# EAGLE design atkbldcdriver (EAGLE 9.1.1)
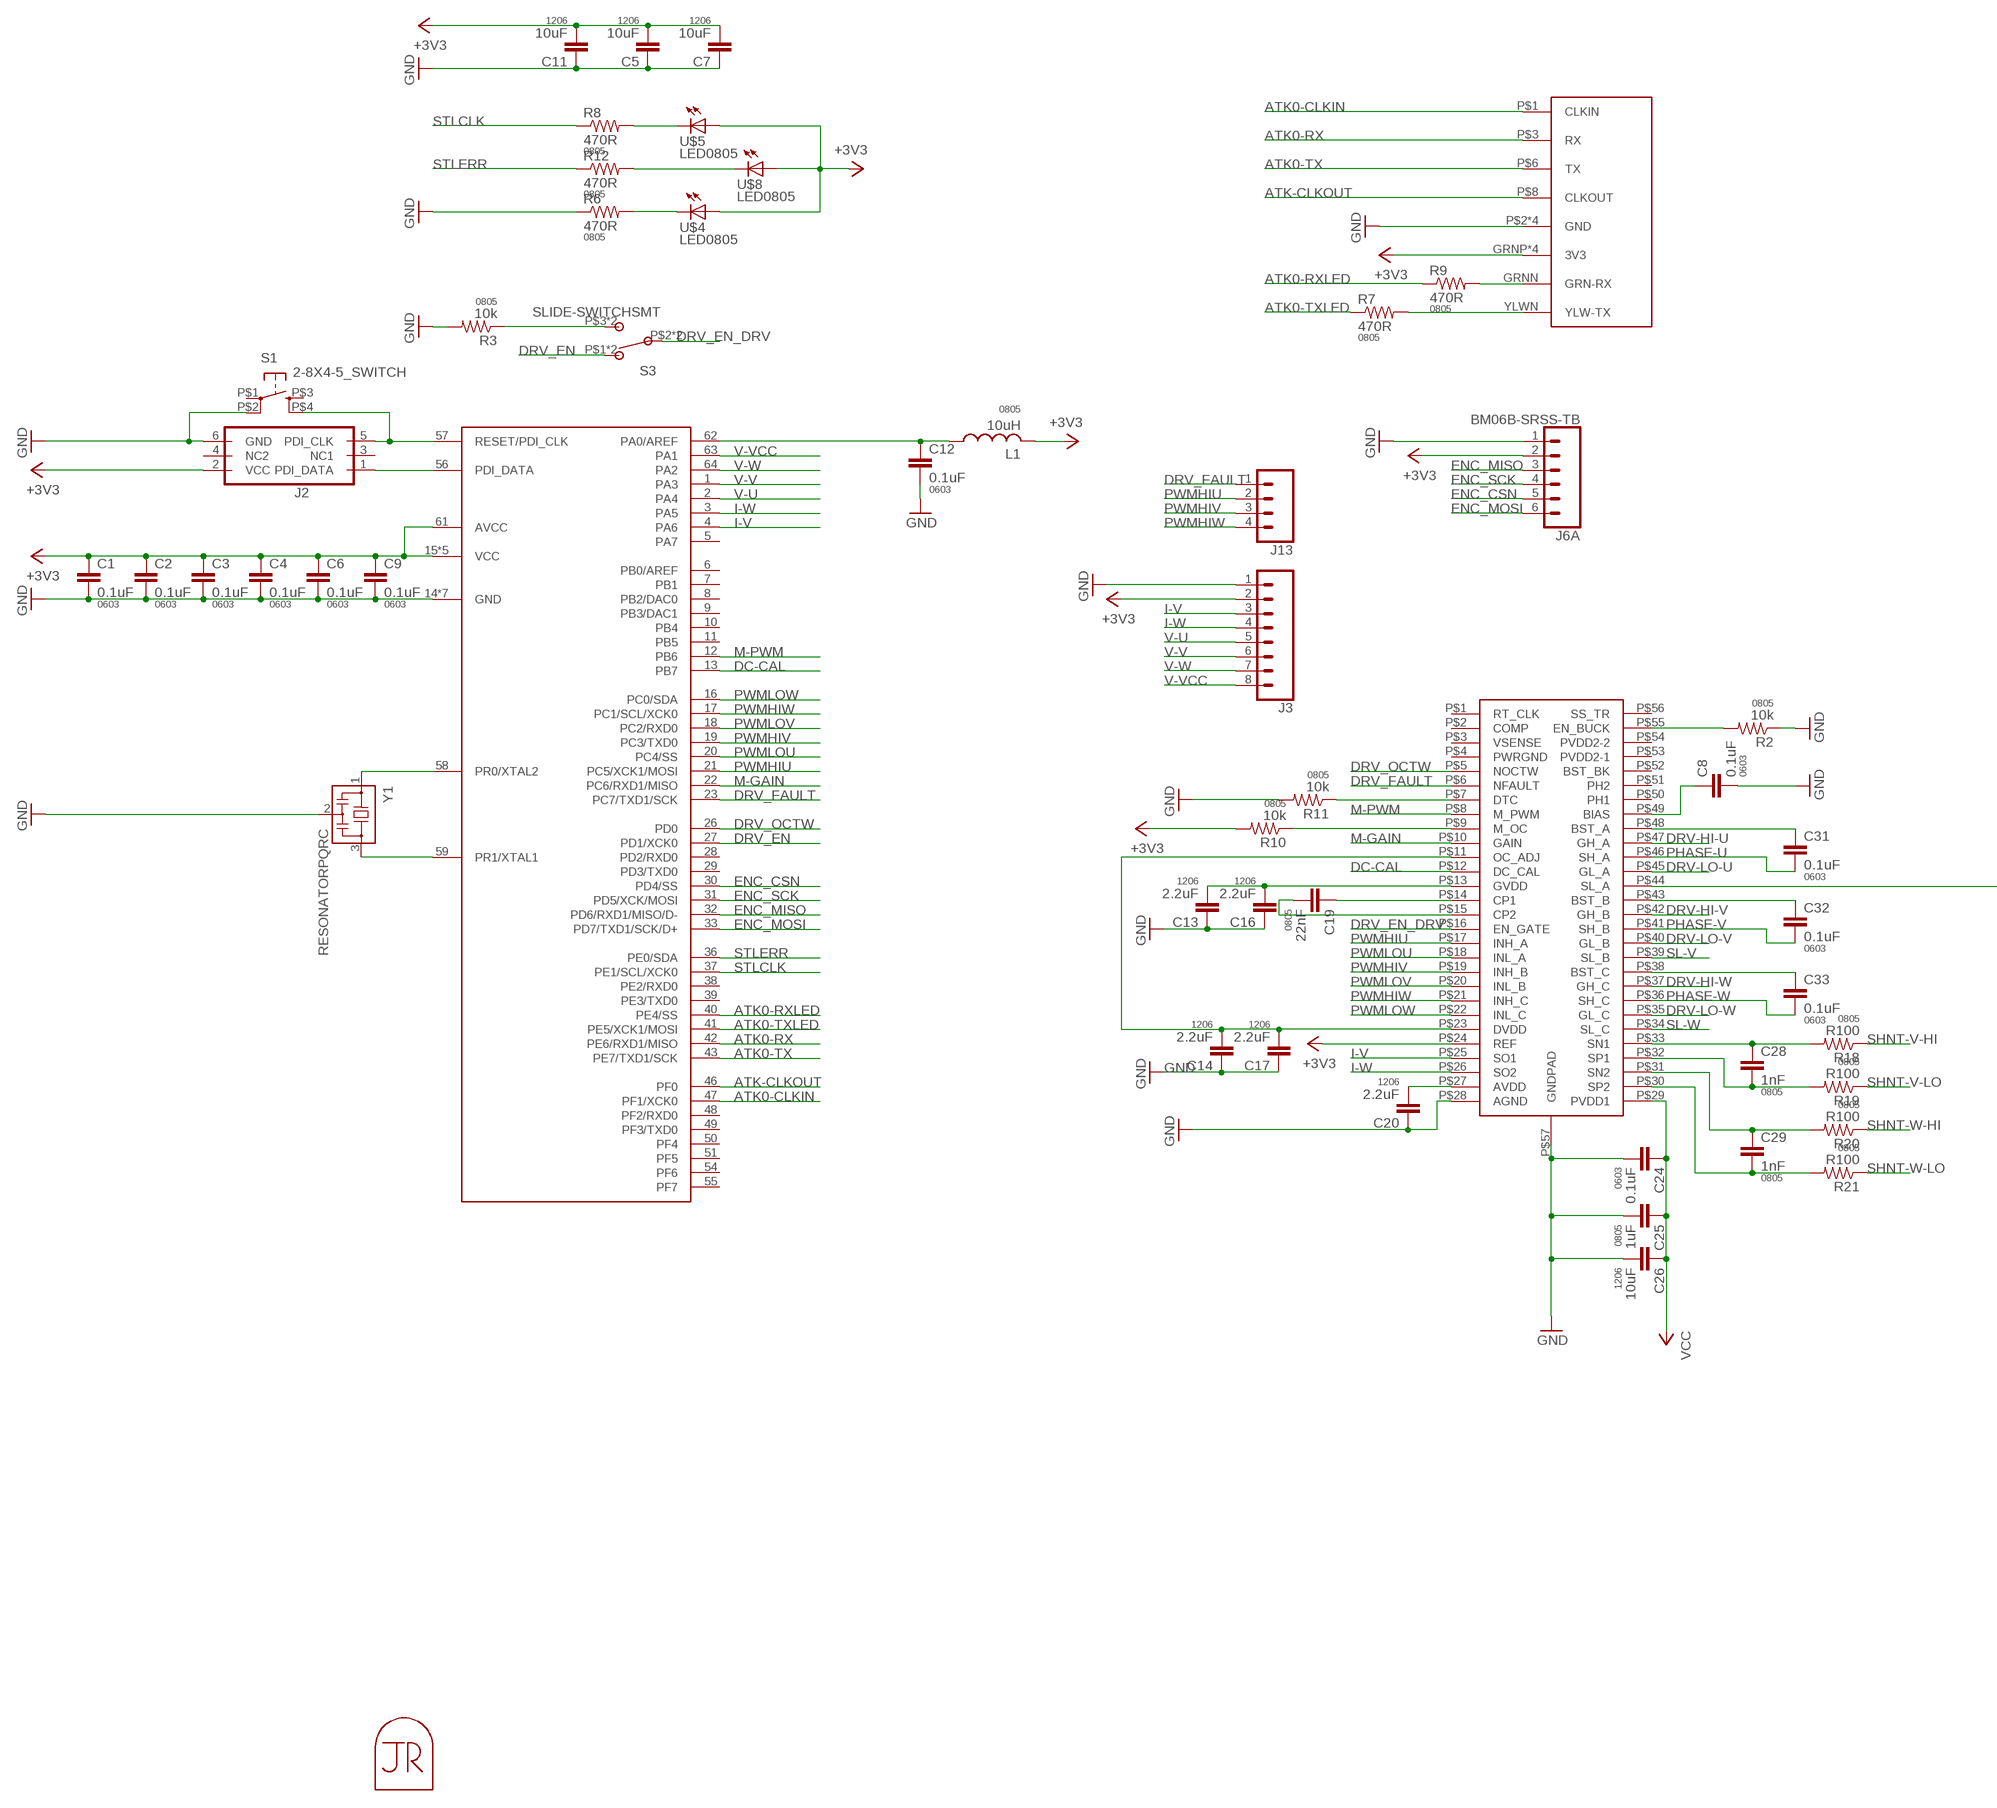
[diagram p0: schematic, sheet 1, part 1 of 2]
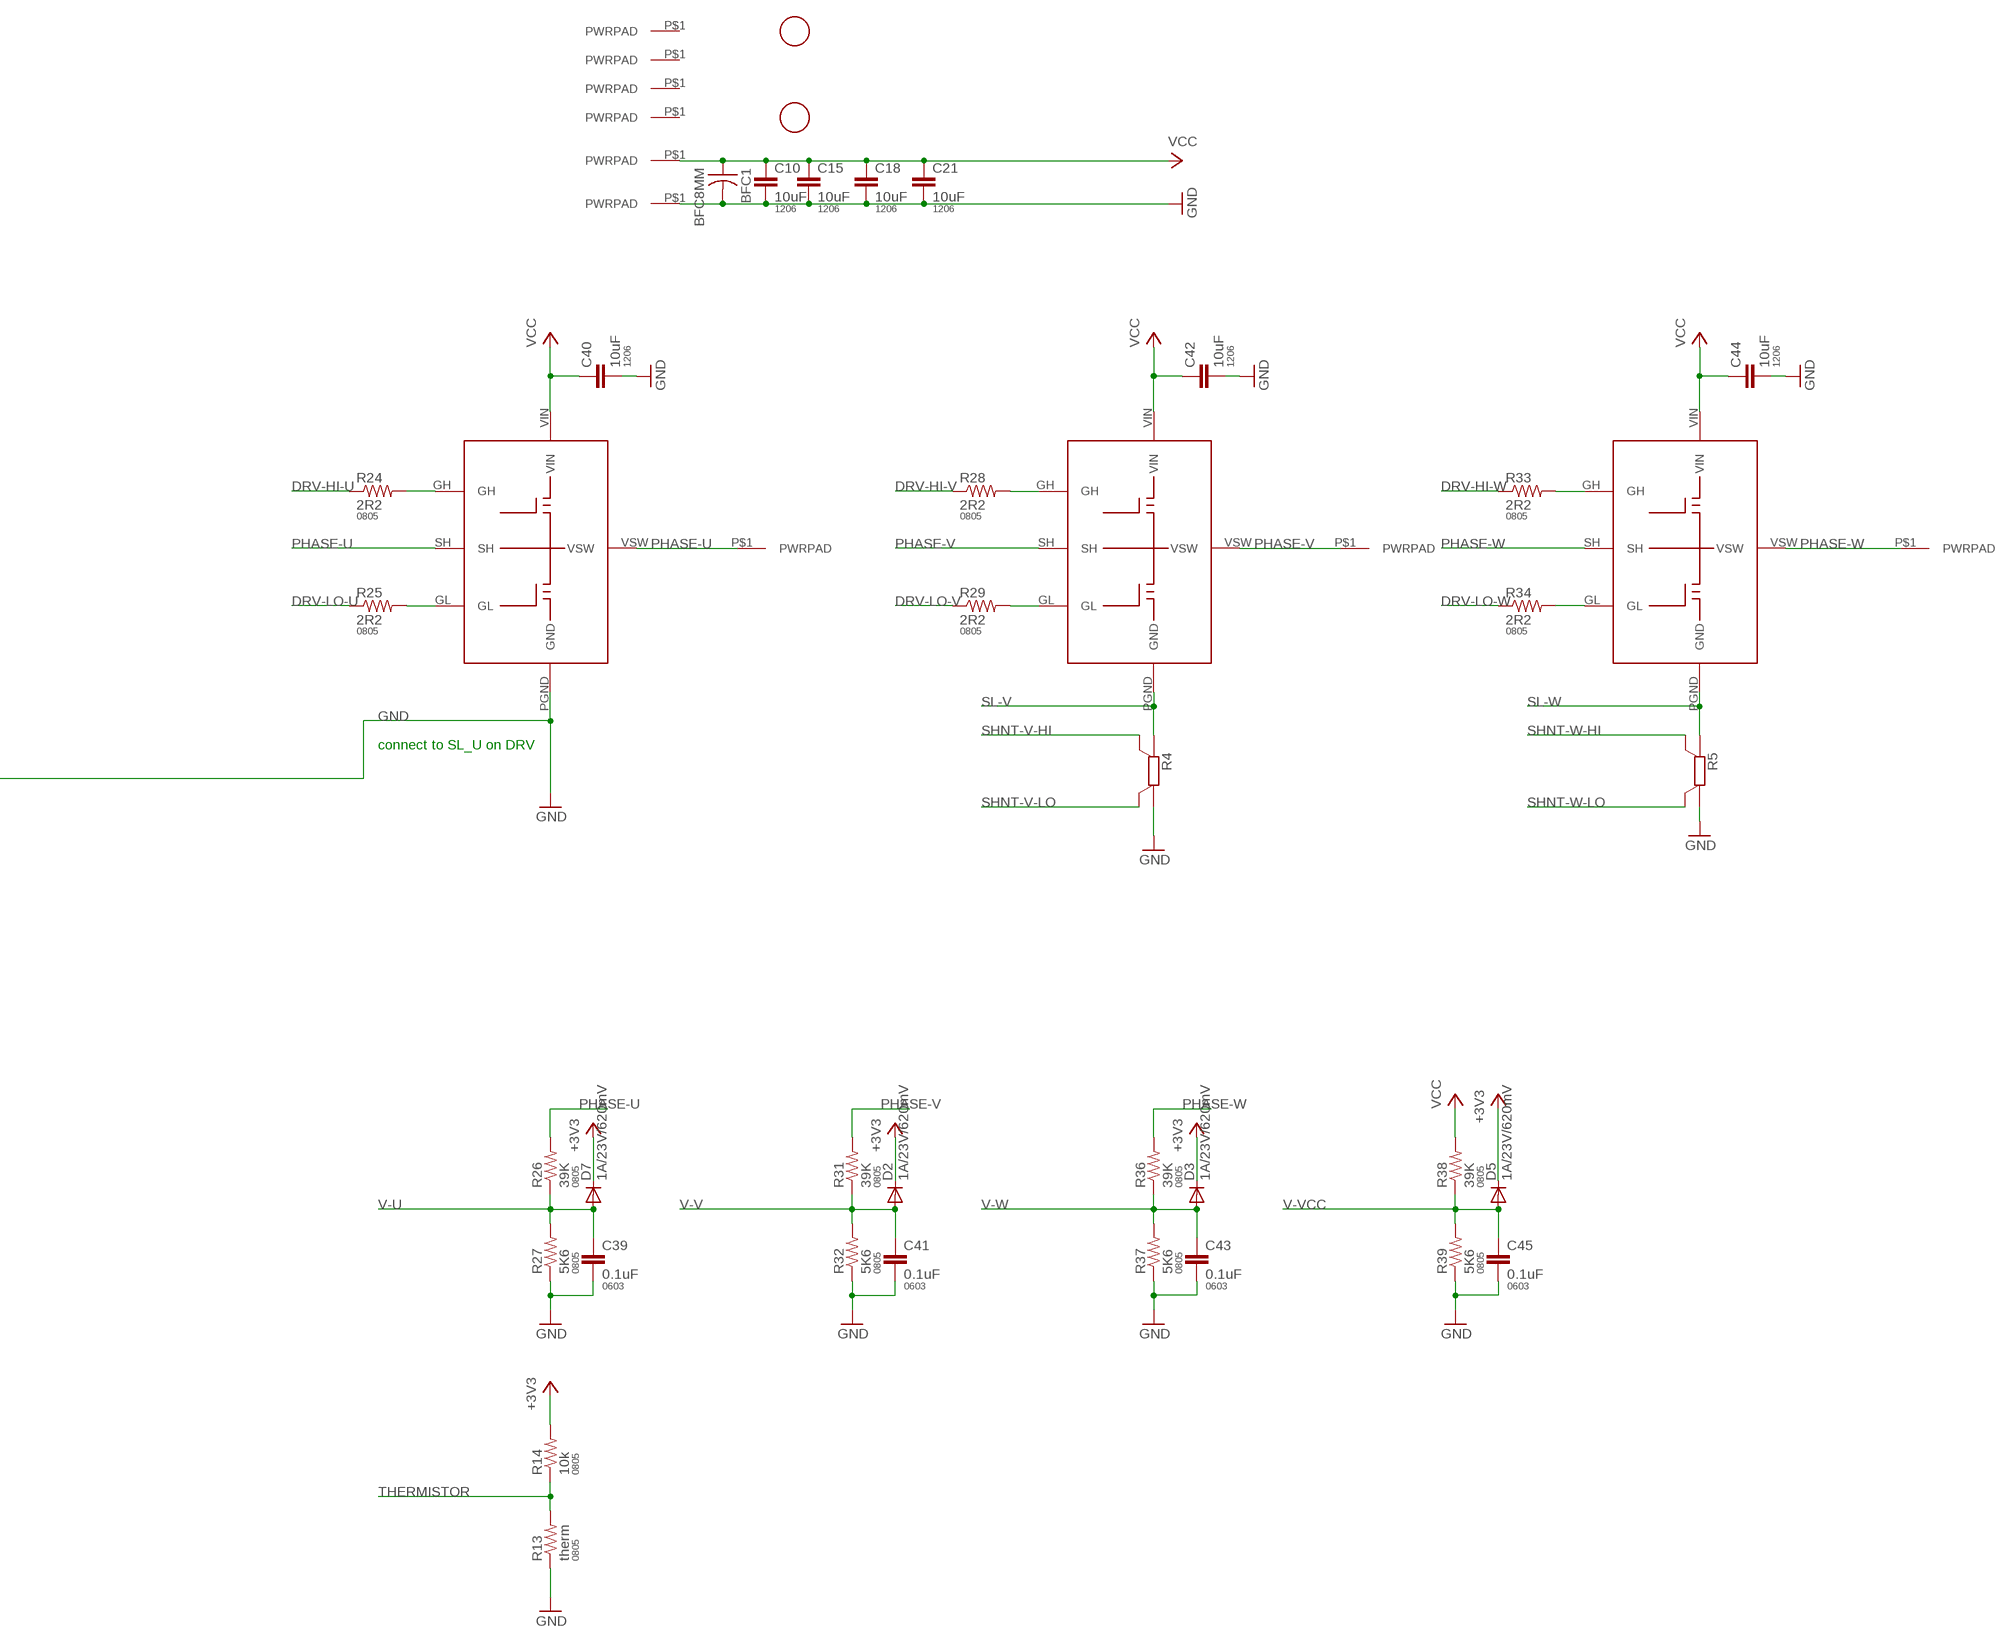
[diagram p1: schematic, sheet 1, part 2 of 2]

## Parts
BFC1  BFC8MM  [BFC-8MM]
C1  0.1uF  CAP0603-CAP  [0603-CAP]
C2  0.1uF  CAP0603-CAP  [0603-CAP]
C3  0.1uF  CAP0603-CAP  [0603-CAP]
C4  0.1uF  CAP0603-CAP  [0603-CAP]
C5  10uF  CAP1206  [1206]
C6  0.1uF  CAP0603-CAP  [0603-CAP]
C7  10uF  CAP1206  [1206]
C8  0.1uF  CAP0603-CAP  [0603-CAP]
C9  0.1uF  CAP0603-CAP  [0603-CAP]
C10  10uF  CAP1206  [1206]
C11  10uF  CAP1206  [1206]
C12  0.1uF  CAP0603-CAP  [0603-CAP]
C13  2.2uF  CAP1206  [1206]
C14  2.2uF  CAP1206  [1206]
C15  10uF  CAP1206  [1206]
C16  2.2uF  CAP1206  [1206]
C17  2.2uF  CAP1206  [1206]
C18  10uF  CAP1206  [1206]
C19  22nF  CAP0805  [0805]
C20  2.2uF  CAP1206  [1206]
C21  10uF  CAP1206  [1206]
C24  0.1uF  CAP0603-CAP  [0603-CAP]
C25  1uF  CAP0805  [0805]
C26  10uF  CAP1206  [1206]
C28  1nF  CAP0805  [0805]
C29  1nF  CAP0805  [0805]
C31  0.1uF  CAP0603-CAP  [0603-CAP]
C32  0.1uF  CAP0603-CAP  [0603-CAP]
C33  0.1uF  CAP0603-CAP  [0603-CAP]
C39  0.1uF  CAP0603-CAP  [0603-CAP]
C40  10uF  CAP1206  [1206]
C41  0.1uF  CAP0603-CAP  [0603-CAP]
C42  10uF  CAP1206  [1206]
C43  0.1uF  CAP0603-CAP  [0603-CAP]
C44  10uF  CAP1206  [1206]
C45  0.1uF  CAP0603-CAP  [0603-CAP]
D2  1A/23V/620mV  DIODEDIODE  [0805-DIODE]
D3  1A/23V/620mV  DIODEDIODE  [0805-DIODE]
D5  1A/23V/620mV  DIODEDIODE  [0805-DIODE]
D7  1A/23V/620mV  DIODEDIODE  [0805-DIODE]
J1  ATK-PHY  [RJ45-LED-RJE7318800XXX]
J2  PDIFEMALE_SMD  [PDI_2X3_SMD]
J3  CONN_08NO_SILK_FEMALE_PTH  [1X08_NO_SILK]
J4  PWRPADM3  [PWRPAD_3-25MM]
J6  BM06B-SRSS-TB  JST_6_PIN_HORIZONTAL  [JST-6-SMD-HORI-1.0MM]
J7  PWRPAD  [PWRPAD_M3-PEM-MOUNT]
J8  PWRPAD  [PWRPAD_M3-PEM-MOUNT]
J9  PWRPAD  [PWRPAD_M3-PEM-MOUNT]
J10  PWRPAD  [PWRPAD_M3-PEM-MOUNT]
J11  PWRPAD  [PWRPAD_M3-PEM-MOUNT]
J12  PWRPADM3  [PWRPAD_3-25MM]
J13  CONN_041X04_NO_SILK  [1X04_NO_SILK]
J14  PWRPADM3  [PWRPAD_3-25MM]
J15  PWRPADM3  [PWRPAD_3-25MM]
L1  10uH  INDUCTOR-0805  [0805]
R2  10k  RESISTOR0805-RES  [0805]
R3  10k  RESISTOR0805-RES  [0805]
R4  R_SHUNT2512  [R2512]
R5  R_SHUNT2512  [R2512]
R6  470R  RESISTOR0805-RES  [0805]
R7  470R  RESISTOR0805-RES  [0805]
R8  470R  RESISTOR0805-RES  [0805]
R9  470R  RESISTOR0805-RES  [0805]
R10  10k  RESISTOR0805-RES  [0805]
R11  10k  RESISTOR0805-RES  [0805]
R12  470R  RESISTOR0805-RES  [0805]
R13  therm  RESISTOR0805-RES  [0805]
R14  10k  RESISTOR0805-RES  [0805]
R18  R100  RESISTOR0805-RES  [0805]
R19  R100  RESISTOR0805-RES  [0805]
R20  R100  RESISTOR0805-RES  [0805]
R21  R100  RESISTOR0805-RES  [0805]
R24  2R2  RESISTOR0805-RES  [0805]
R25  2R2  RESISTOR0805-RES  [0805]
R26  39K  RESISTOR0805-RES  [0805]
R27  5K6  RESISTOR0805-RES  [0805]
R28  2R2  RESISTOR0805-RES  [0805]
R29  2R2  RESISTOR0805-RES  [0805]
R31  39K  RESISTOR0805-RES  [0805]
R32  5K6  RESISTOR0805-RES  [0805]
R33  2R2  RESISTOR0805-RES  [0805]
R34  2R2  RESISTOR0805-RES  [0805]
R36  39K  RESISTOR0805-RES  [0805]
R37  5K6  RESISTOR0805-RES  [0805]
R38  39K  RESISTOR0805-RES  [0805]
R39  5K6  RESISTOR0805-RES  [0805]
S1  2-8X4-5_SWITCH  [TACT-SWITCH-KMR6]
S3  SLIDE-SWITCHSMT  [SLIDESWITCH-CL-SB-22A]
U1  ATXMEGA_A3UQFN  [QFN-64-9X9MM]
U2  DRV8302  [HTSSOP-56]
U$1  FIDUCIAL  [FIDUCIAL_1MM]
U$3  FIDUCIAL  [FIDUCIAL_1MM]
U$4  LED0805  [LED0805]
U$5  LED0805  [LED0805]
U$8  LED0805  [LED0805]
U$9  INTEGRATED_HALF-CSD88599SON  [SON-5X6]
U$10  INTEGRATED_HALF-CSD88599SON  [SON-5X6]
U$11  INTEGRATED_HALF-CSD88599SON  [SON-5X6]
U$14  JRTOMBSTONE  [JRTOMBSTONE]
Y1  RESONATORPQRC  [RES_PRQC]

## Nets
+3V3: C1.1 C2.1 C3.1 C4.1 C5.2 C6.1 C7.2 C9.1 C11.2 D2.2(C) D3.2(C) D5.2(C) D7.2(C) J1.GRNP(3V3) J1.P$4(3V3) J1.P$5(3V3) J1.YLWP(3V3) J2.2(VCC) J3.2 J6.2 L1.2 R10.2 R14.2 U1.15(VCC) U1.25(VCC) U1.35(VCC) U1.45(VCC) U1.53(VCC) U1.61(AVCC) U2.P$24(REF) U$4.1(A) U$5.1(A) U$8.1(A)
ATK0-CLKIN: J1.P$1(CLKIN) U1.47(PF1/XCK0)
ATK0-RX: J1.P$3(RX) U1.42(PE6/RXD1/MISO)
ATK0-RXLED: R9.1 U1.40(PE4/SS)
ATK0-TX: J1.P$6(TX) U1.43(PE7/TXD1/SCK)
ATK0-TXLED: R7.1 U1.41(PE5/XCK1/MOSI)
ATK-CLKOUT: J1.P$8(CLKOUT) U1.46(PF0)
CP1: C19.1 U2.P$14(CP1)
CP2: C19.2 U2.P$15(CP2)
DC-CAL: U1.13(PB7) U2.P$12(DC_CAL)
DRV-HI-U: R24.1 U2.P$47(GH_A)
DRV-HI-V: R28.1 U2.P$42(GH_B)
DRV-HI-W: R33.1 U2.P$37(GH_C)
DRV-LO-U: R25.1 U2.P$45(GL_A)
DRV-LO-V: R29.1 U2.P$40(GL_B)
DRV-LO-W: R34.1 U2.P$35(GL_C)
DRV_EN: S3.P$1 S3.P$4 U1.27(PD1/XCK0)
DRV_EN_DRV: S3.P$2 S3.P$5 U2.P$16(EN_GATE)
DRV_FAULT: J13.1 U1.23(PC7/TXD1/SCK) U2.P$6(NFAULT)
DRV_OCTW: U1.26(PD0) U2.P$5(NOCTW)
ENC_CSN: J6.5 U1.30(PD4/SS)
ENC_MISO: J6.3 U1.32(PD6/RXD1/MISO/D-)
ENC_MOSI: J6.6 U1.33(PD7/TXD1/SCK/D+)
ENC_SCK: J6.4 U1.31(PD5/XCK/MOSI)
GND: BFC1.P$2 C1.2 C2.2 C3.2 C4.2 C5.1 C6.2 C7.1 C8.2 C9.2 C10.2 C11.1 C12.2 C13.1 C14.1 C15.2 C16.1 C17.1 C18.2 C20.1 C21.2 C24.2 C25.2 C26.2 C39.2 C40.2 C41.2 C42.2 C43.2 C44.2 C45.2 J1.P$2(GND) J1.P$7(GND) J1.SHDL1(GND) J1.SHDL2(GND) J2.6(GND) J3.1 J6.1 J9.P$1(PWRPAD) R2.1 R3.2 R4.A R5.A R6.1 R11.2 R13.1 R27.1 R32.1 R37.1 R39.1 S1.P$2(P1) U1.14(GND) U1.24(GND) U1.34(GND) U1.44(GND) U1.52(GND) U1.60(GND) U1.P$1(GND) U2.P$28(AGND) U2.P$44(SL_A) U2.P$57(GNDPAD) U$9.PGND(GND) Y1.2
I-V: J3.3 U1.4(PA6) U2.P$25(SO1)
I-W: J3.4 U1.3(PA5) U2.P$26(SO2)
M-GAIN: U1.22(PC6/RXD1/MISO) U2.P$10(GAIN)
M-PWM: U1.12(PB6) U2.P$8(M_PWM)
N$1: J1.YLWN(YLW-TX) R7.2
N$2: R25.2 U$9.GL
N$3: R24.2 U$9.GH
N$4: R28.2 U$10.GH
N$5: R33.2 U$11.GH
N$6: R34.2 U$11.GL
N$7: C33.1 U2.P$38(BST_C)
N$8: C32.1 U2.P$43(BST_B)
N$9: C31.1 U2.P$48(BST_A)
N$10: R2.2 U2.P$55(EN_BUCK)
N$11: C20.2 U2.P$27(AVDD)
N$12: U1.58(PR0/XTAL2) Y1.1
N$13: C28.1 R18.2 U2.P$33(SN1)
N$14: C28.2 R19.2 U2.P$32(SP1)
N$15: C29.1 R20.2 U2.P$31(SN2)
N$16: C29.2 R21.2 U2.P$30(SP2)
N$17: U1.59(PR1/XTAL1) Y1.3
N$18: C13.2 C16.2 U2.P$13(GVDD)
N$19: C8.1 U2.P$49(BIAS)
N$20: C14.2 C17.2 U2.P$11(OC_ADJ) U2.P$23(DVDD)
N$21: R11.1 U2.P$7(DTC)
N$22: J1.GRNN(GRN-RX) R9.2
N$23: R12.2 U$8.2(C)
N$24: R29.2 U$10.GL
N$25: R10.1 U2.P$9(M_OC)
N$26: R3.1 S3.P$3 S3.P$6
N$27: J2.1(PDI_DATA) U1.56(PDI_DATA)
N$28: J2.5(PDI_CLK) S1.P$4(S1) U1.57(RESET/PDI_CLK)
N$34: C12.1 L1.1 U1.62(PA0/AREF)
N$35: R6.2 U$4.2(C)
N$36: R8.2 U$5.2(C)
PHASE-U: C31.2 J7.P$1(PWRPAD) R26.2 U2.P$46(SH_A) U$9.SH U$9.VSW
PHASE-V: C32.2 J10.P$1(PWRPAD) R31.2 U2.P$41(SH_B) U$10.SH U$10.VSW
PHASE-W: C33.2 J11.P$1(PWRPAD) R36.2 U2.P$36(SH_C) U$11.SH U$11.VSW
PWMHIU: J13.2 U1.21(PC5/XCK1/MOSI) U2.P$17(INH_A)
PWMHIV: J13.3 U1.19(PC3/TXD0) U2.P$19(INH_B)
PWMHIW: J13.4 U1.17(PC1/SCL/XCK0) U2.P$21(INH_C)
PWMLOU: U1.20(PC4/SS) U2.P$18(INL_A)
PWMLOV: U1.18(PC2/RXD0) U2.P$20(INL_B)
PWMLOW: U1.16(PC0/SDA) U2.P$22(INL_C)
SHNT-V-HI: R4.SB R18.1
SHNT-V-LO: R4.SA R19.1
SHNT-W-HI: R5.SB R20.1
SHNT-W-LO: R5.SA R21.1
SL-V: R4.B U2.P$39(SL_B) U$10.PGND(GND)
SL-W: R5.B U2.P$34(SL_C) U$11.PGND(GND)
STLCLK: R8.1 U1.37(PE1/SCL/XCK0)
STLERR: R12.1 U1.36(PE0/SDA)
THERMISTOR: R13.2 R14.1
V-U: C39.1 D7.1(A) J3.5 R26.1 R27.2 U1.2(PA4)
V-V: C41.1 D2.1(A) J3.6 R31.1 R32.2 U1.1(PA3)
V-VCC: C45.1 D5.1(A) J3.8 R38.1 R39.2 U1.63(PA1)
V-W: C43.1 D3.1(A) J3.7 R36.1 R37.2 U1.64(PA2)
VCC: BFC1.P$1 C10.1 C15.1 C18.1 C21.1 C24.1 C25.1 C26.1 C40.1 C42.1 C44.1 J8.P$1(PWRPAD) R38.2 U2.P$29(PVDD1) U$9.VIN U$10.VIN U$11.VIN
Unconnected: J2.3(NC1) J2.4(NC2) J4.P$1(PWRPAD) J6.M1 J6.M2 J12.P$1(PWRPAD) J14.P$1(PWRPAD) J15.P$1(PWRPAD) S1.P$1(P) S1.P$3(S) U1.5(PA7) U1.6(PB0/AREF) U1.7(PB1) U1.8(PB2/DAC0) U1.9(PB3/DAC1) U1.10(PB4) U1.11(PB5) U1.28(PD2/RXD0) U1.29(PD3/TXD0) U1.38(PE2/RXD0) U1.39(PE3/TXD0) U1.48(PF2/RXD0) U1.49(PF3/TXD0) U1.50(PF4) U1.51(PF5) U1.54(PF6) U1.55(PF7) U2.P$1(RT_CLK) U2.P$2(COMP) U2.P$3(VSENSE) U2.P$4(PWRGND) U2.P$50(PH1) U2.P$51(PH2) U2.P$52(BST_BK) U2.P$53(PVDD2-1) U2.P$54(PVDD2-2) U2.P$56(SS_TR)

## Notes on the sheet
- connect to SL_U on DRV

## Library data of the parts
BFC1 = power:BFC
C1-C4 C6 C8 C9 C12 C24 C31-C33 C39 C41 C43 C45 = borkedlabs-passives:CAP: Capacitor; PACKAGE: 0603
C5 C7 C10 C11 C13-C18 C20 C21 C26 C40 C42 C44 = borkedlabs-passives:CAP: Capacitor; PACKAGE: 1206
C19 C25 C28 C29 = borkedlabs-passives:CAP: Capacitor; PACKAGE: 0805
D2 D3 D5 D7 = passives:DIODE: DIODE
J1 = connector:ATK-PHY
J2 = microcontrollers:PDI: Multi connection point. Often used as Generic Header-pin footprint for 0.1 inch spaced/style header connections You can populate with any combo of single row headers, but if you'd like an exact match, check these: Header - 2x3 (Male, 0.1") (PRT-12807) Header - 2x3 (Female, 0.1") (PRT-13010) 2x3 Pin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; PROD_ID: CONN-11290
J3 = SparkFun-Connectors:CONN_08: Multi connection point. Often used as Generic Header-pin footprint for 0.1 inch spaced/style header connections On any of the 0.1 inch spaced packages, you can populate with these: Break Away Headers - Straight (PRT-00116) Break Away Male Headers - Right Angle (PRT-00553) Female Headers (PRT-00115)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; PROD_ID: CONN-08438
J4 J7-J12 J14 J15 = power:PWRPAD
J6 = SparkFun-Connectors:JST_6_PIN_HORIZONTAL: JST 6 pin horizontal connector JST-SH type. Here is the connector we sell at SparkFun: name (XXX-00000) Datasheet It was used on these SparkFun products: name (XXX-00000) name (XXX-00000); PROD_ID: XXX-00000
J13 = SparkFun-Connectors:CONN_04: Multi connection point. Often used as Generic Header-pin footprint for 0.1 inch spaced/style header connections On any of the 0.1 inch spaced packages, you can populate with these: Break Away Headers - Straight (PRT-00116) Break Away Male Headers - Right Angle (PRT-00553) Female Headers (PRT-00115)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; PROD_ID: CONN-09696
L1 = borkedlabs-passives:INDUCTOR; PACKAGE: 0805
R2 R3 R6-R14 R18-R21 R24-R29 R31-R34 R36-R39 = borkedlabs-passives:RESISTOR: Resistor; PACKAGE: 0805
R4 R5 = power:R_SHUNT: Resistor Basic schematic elements and footprints for 0603, 1206, and PTH resistors.
S1 = fab:2-8X4-5_SWITCH
S3 = fab:SLIDE-SWITCH: SMD slide-switch AYZ0102AGRLC as found in the fablab inventory. Includes the mounting holes. Made by Zaerc.
U1 = microcontrollers:ATXMEGA_A3U
U2 = power:DRV8302
U$1 U$3 = connector:FIDUCIAL: For use by pick and place machines to calibrate the vision/machine, 1mm
U$4 U$5 U$8 = lights:LED: LED
U$9-U$11 = power:INTEGRATED_HALF-CSD88599
U$14 = connector:JRTOMBSTONE
Y1 = passives:RESONATOR

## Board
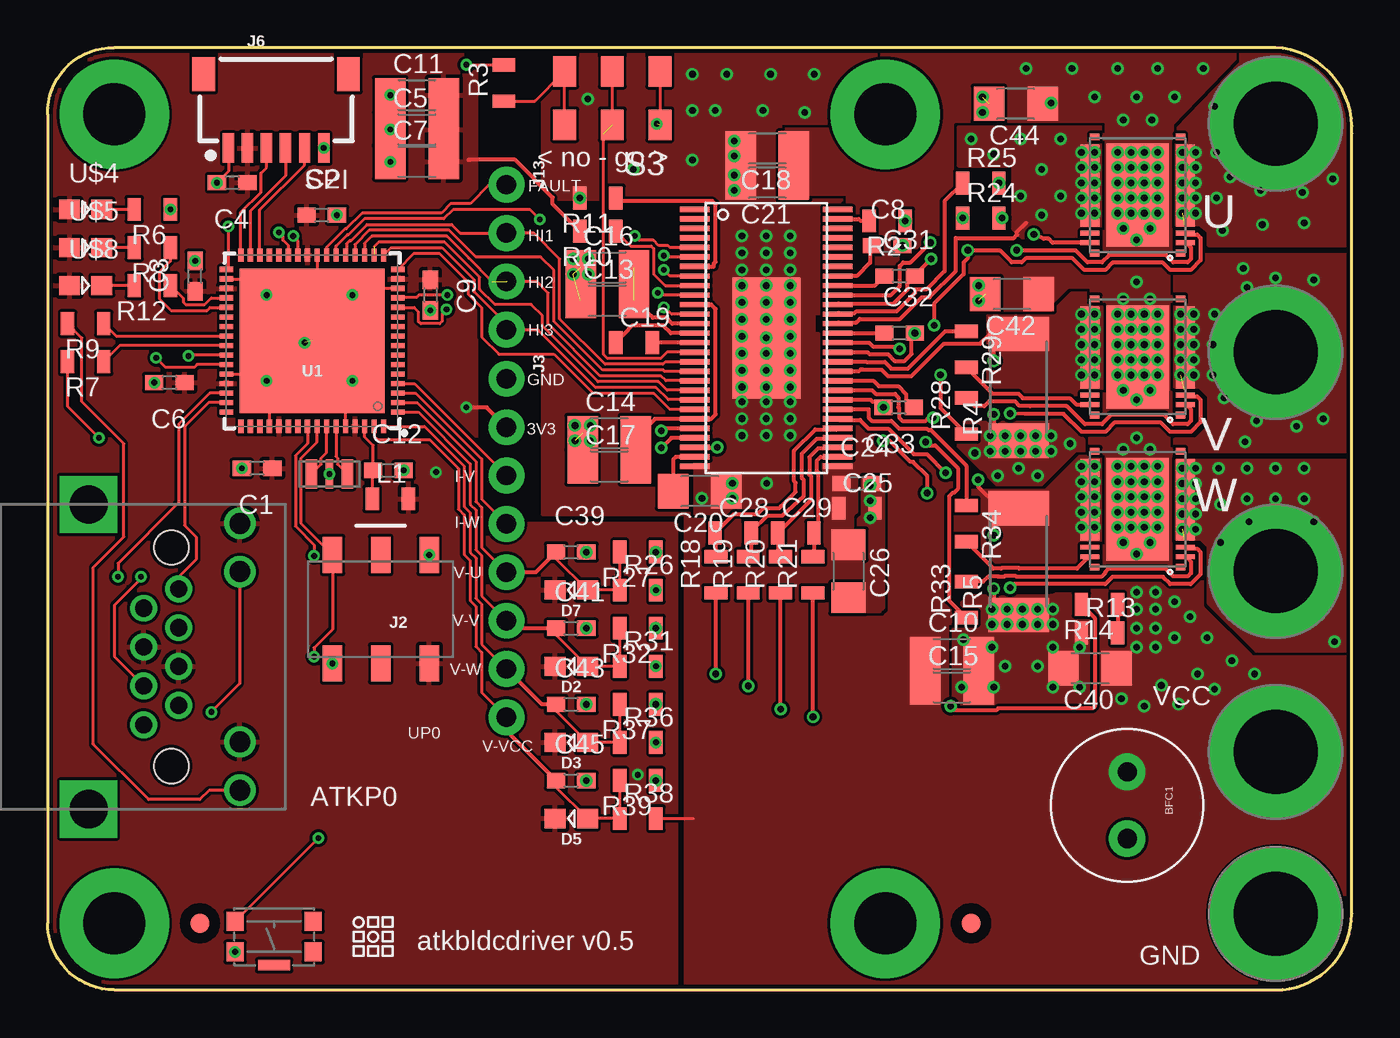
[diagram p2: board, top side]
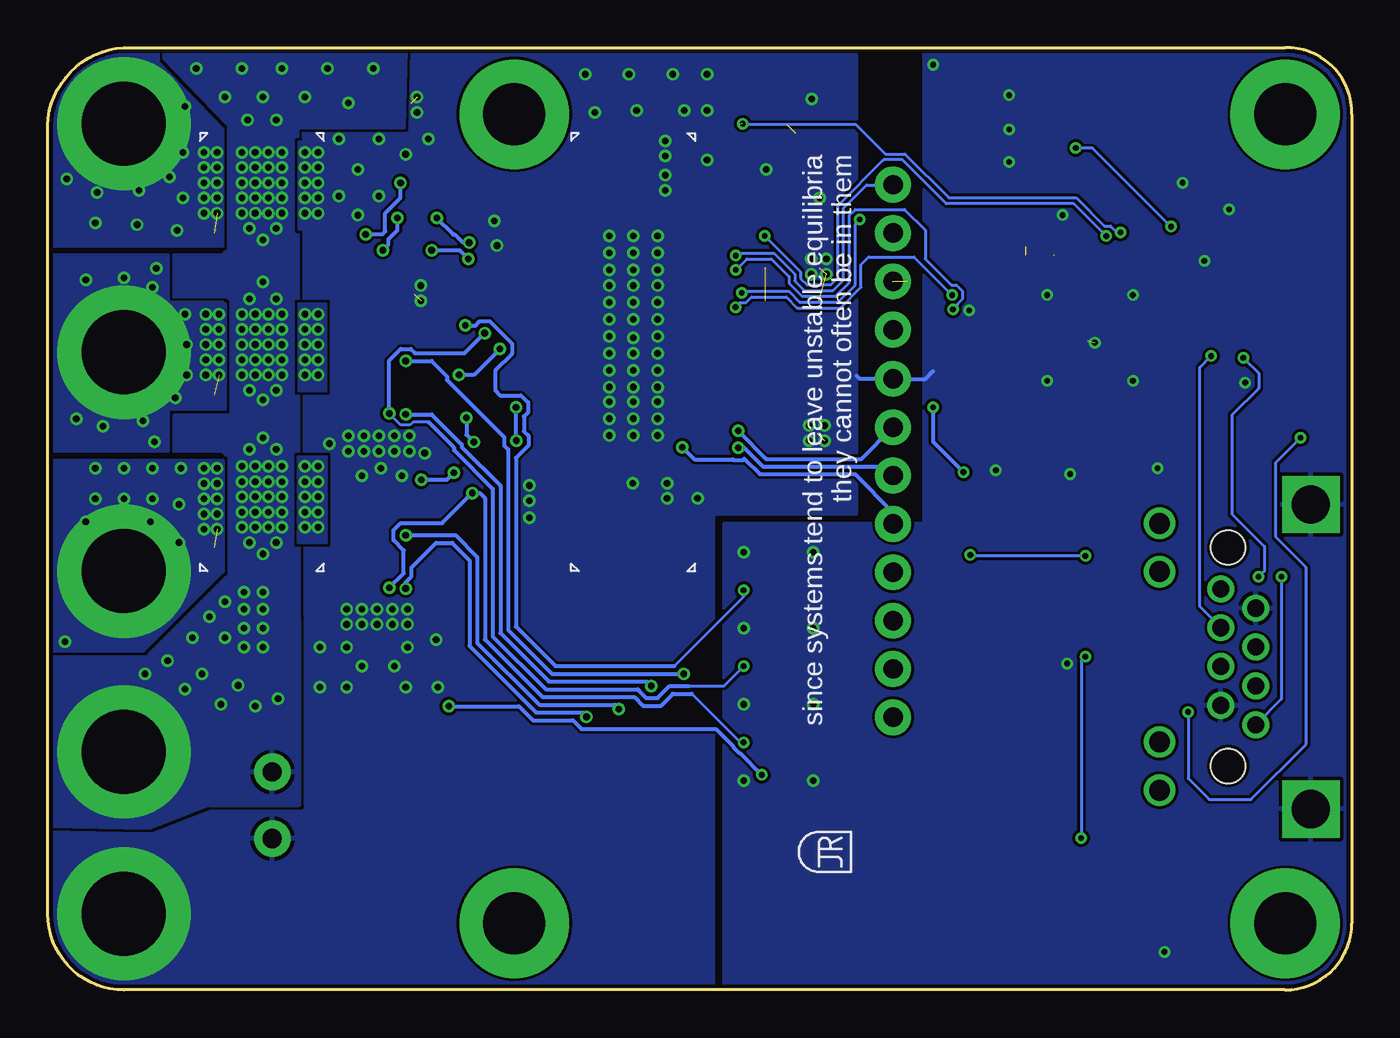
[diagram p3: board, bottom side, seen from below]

Size 68.5 x 49.5 mm. Coordinates in mm from the lower left corner, seen from the top.
Outline: 0,46 arc-92 3.5,49.5 64.5,49.5 arc-90 68.5,45 68.5,4 arc-90 64.5,0 3.5,0 arc-90 0,3.5 0,46
Copper layers (1*16): Top 0.035mm / dielectric 1.5mm / Bottom 0.035mm
Design rules "default *": minimum track width 6mil, minimum drill 0.3mm, track to track 6mil, track to pad 6mil, pad to pad 6mil, via to via 6mil, smd to smd 6mil, copper to edge 8mil, drill to drill 8mil, minimum pad ring 10mil, minimum via ring 6mil, stop-mask expansion 4mil, vias tented up to drill 20mil, thermal gap 8mil

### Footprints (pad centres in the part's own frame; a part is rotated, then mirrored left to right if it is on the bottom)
BFC-8MM = drill 1 pad 1.93: P$1 -1.75,0; P$2 1.75,0
0603-CAP = smd 0.96 x 0.8: 1 -0.8,0; 2 0.8,0
1206 = smd 1.6 x 1.8: 1 -1.4,0; 2 1.4,0
0805 = smd 0.7 x 1.2: 1 -0.95,0; 2 0.95,0
0805-DIODE = smd 1.1 x 1: 1 -0.85,0; 2 0.85,0
RJ45-LED-RJE7318800XXX = drill 1.1: GRNN 7.01,3.6; GRNP 4.47,3.6; YLWN -4.47,3.6; YLWP -7.01,3.6 | drill 0.9: P$1 -3.57,0.38; P$2 -2.55,-1.45; P$3 -1.53,0.38; P$4 -0.51,-1.45; P$5 0.51,0.38; P$6 1.53,-1.45; P$7 2.55,0.38; P$8 3.57,-1.45 | drill 2 square: SHDL1 -8,-4.35; SHDL2 8,-4.35 | hole 1.8: -5.74,0; 5.74,0
PDI_2X3_SMD = smd 1.02 x 1.9: 1 -2.54,-2.85; 2 -2.54,2.85; 3 0,-2.85; 4 0,2.85; 5 2.54,-2.85; 6 2.54,2.85
1X08_NO_SILK = drill 1.016 pad 1.88: 1 0,0; 2 2.54,0; 3 5.08,0; 4 7.62,0; 5 10.16,0; 6 12.7,0; 7 15.24,0; 8 17.78,0
PWRPAD_3-25MM = drill 3.25 pad 5.75: P$1 0,0
JST-6-SMD-HORI-1.0MM = smd 0.6 x 1.55: 1 -2.5,-4.775; 2 -1.5,-4.775; 3 -0.5,-4.775; 4 0.5,-4.775; 5 1.5,-4.775; 6 2.5,-4.775 | smd 1.2 x 1.8: M1 -3.8,-0.9; M2 3.8,-0.9
PWRPAD_M3-PEM-MOUNT = drill 4.4 pad 7: P$1 0,0
1X04_NO_SILK = drill 1.016 pad 1.88: 1 0,0; 2 2.54,0; 3 5.08,0; 4 7.62,0
R2512 = smd 1.8 x 3.2: A -2.8,0; B 2.8,0 | smd 0.5 x 0.5: SA -1.414,1.3; SB 1.386,1.3
TACT-SWITCH-KMR6 = smd 0.9 x 1: P$1 -2.05,0.8; P$2 2.05,0.8; P$3 -2.05,-0.8; P$4 2.05,-0.8 | smd 1.7 x 0.55: P$5 0,1.5
SLIDESWITCH-CL-SB-22A = smd 1.2 x 1.6: P$1 -2.5,1.4; P$2 0,1.4; P$3 2.5,1.4; P$4 -2.5,-1.4; P$5 0,-1.4; P$6 2.5,-1.4
QFN-64-9X9MM = smd 0.7 x 0.275: 1 -4.5,3.75; 2 -4.5,3.25; 3 -4.5,2.75; 4 -4.5,2.25; 5 -4.5,1.75; 6 -4.5,1.25; 7 -4.5,0.75; 8 -4.5,0.25; 9 -4.5,-0.25; 10 -4.5,-0.75; 11 -4.5,-1.25; 12 -4.5,-1.75; 13 -4.5,-2.25; 14 -4.5,-2.75; 15 -4.5,-3.25; 16 -4.5,-3.75; 33 4.5,-3.75; 34 4.5,-3.25; 35 4.5,-2.75; 36 4.5,-2.25; 37 4.5,-1.75; 38 4.5,-1.25; 39 4.5,-0.75; 40 4.5,-0.25; 41 4.5,0.25; 42 4.5,0.75; 43 4.5,1.25; 44 4.5,1.75; 45 4.5,2.25; 46 4.5,2.75; 47 4.5,3.25; 48 4.5,3.75 | smd 0.275 x 0.7: 17 -3.75,-4.5; 18 -3.25,-4.5; 19 -2.75,-4.5; 20 -2.25,-4.5; 21 -1.75,-4.5; 22 -1.25,-4.5; 23 -0.75,-4.5; 24 -0.25,-4.5; 25 0.25,-4.5; 26 0.75,-4.5; 27 1.25,-4.5; 28 1.75,-4.5; 29 2.25,-4.5; 30 2.75,-4.5; 31 3.25,-4.5; 32 3.75,-4.5; 49 3.75,4.5; 50 3.25,4.5; 51 2.75,4.5; 52 2.25,4.5; 53 1.75,4.5; 54 1.25,4.5; 55 0.75,4.5; 56 0.25,4.5; 57 -0.25,4.5; 58 -0.75,4.5; 59 -1.25,4.5; 60 -1.75,4.5; 61 -2.25,4.5; 62 -2.75,4.5; 63 -3.25,4.5; 64 -3.75,4.5 | smd 7.6 x 7.6: P$1 0,0
HTSSOP-56 = smd 1.549 x 0.279: P$1 -3.75,6.75; P$2 -3.75,6.25; P$3 -3.75,5.75; P$4 -3.75,5.25; P$5 -3.75,4.75; P$6 -3.75,4.25; P$7 -3.75,3.75; P$8 -3.75,3.25; P$9 -3.75,2.75; P$10 -3.75,2.25; P$11 -3.75,1.75; P$12 -3.75,1.25; P$13 -3.75,0.75; P$14 -3.75,0.25; P$15 -3.75,-0.25; P$16 -3.75,-0.75; P$17 -3.75,-1.25; P$18 -3.75,-1.75; P$19 -3.75,-2.25; P$20 -3.75,-2.75; P$21 -3.75,-3.25; P$22 -3.75,-3.75; P$23 -3.75,-4.25; P$24 -3.75,-4.75; P$25 -3.75,-5.25; P$26 -3.75,-5.75; P$27 -3.75,-6.25; P$28 -3.75,-6.75; P$29 3.75,-6.75; P$30 3.75,-6.25; P$31 3.75,-5.75; P$32 3.75,-5.25; P$33 3.75,-4.75; P$34 3.75,-4.25; P$35 3.75,-3.75; P$36 3.75,-3.25; P$37 3.75,-2.75; P$38 3.75,-2.25; P$39 3.75,-1.75; P$40 3.75,-1.25; P$41 3.75,-0.75; P$42 3.75,-0.25; P$43 3.75,0.25; P$44 3.75,0.75; P$45 3.75,1.25; P$46 3.75,1.75; P$47 3.75,2.25; P$48 3.75,2.75; P$49 3.75,3.25; P$50 3.75,3.75; P$51 3.75,4.25; P$52 3.75,4.75; P$53 3.75,5.25; P$54 3.75,5.75; P$55 3.75,6.25; P$56 3.75,6.75 | smd 3.581 x 6.35: P$57 0,0
FIDUCIAL_1MM = smd 1 x 1: 1 0,0
LED0805 = smd 1.1 x 1: 1 -0.85,0; 2 0.85,0
SON-5X6 = smd 1 x 0.25: GH -2.5,2.5; GL 2.5,2.5; NC 2.5,2; SH -2.5,2 | smd 0.5 x 0.35: M1 -2.25,3.05; M2 2.25,3.05; M3 -2.25,-3.05; M4 2.25,-3.05 | smd 1 x 4.3: PGND 2.5,-0.5; VSW -2.5,-0.5 | smd 3.3 x 5.4: VIN 0,0
RES_PRQC = smd 0.6 x 1.5: 1 -0.95,0; 3 0.95,0 | smd 0.4 x 1.5: 2 0,0

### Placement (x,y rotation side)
BFC1  56.7,9.7 270 top
C1  11,27.4 180 top
C2  14.4,40.7 0 top
C3  7.75,37.5 90 top
C4  9.7,42.4 180 top
C5  19.4,45.2 0 top
C6  6.4,31.9 180 top
C7  19.4,43.5 0 top
C8  44.1,39.1 0 top
C9  20.1,36.5 270 top
C10  47.5,17.65 0 top
C11  19.4,47 0 top
C12  17.9,27.3 0 top
C13  29.4,36.2 0 top
C14  29.5,29.25 0 top
C15  47.5,15.9 0 top
C16  29.4,37.95 0 top
C17  29.5,27.5 0 top
C18  37.8,44.2 180 top
C19  30.8,34 0 top
C20  34.25,26.2 180 top
C21  37.8,42.4 180 top
C24  42.5,26.6 0 top
C25  42.5,25.3 0 top
C26  42.06,21.99 270 top
C28  36,24 0 top
C29  39.3,24 0 top
C31  44.75,37.5 0 top
C32  44.75,34.5 0 top
C33  44.7,30.6 180 top
C39  27.5,23 0 top
C40  54.75,16.9 180 top
C41  27.5,19 0 top
C42  50.65,36.55 180 top
C43  27.5,15 0 top
C44  50.85,46.55 180 top
C45  27.5,11 0 top
D2  27.5,17 180 top
D3  27.5,13 180 top
D5  27.5,9 180 top
D7  27.5,21 180 top
J1  6.5,17.5 270 top
J2  17.5,20 180 top
J3  24.1,32.1 270 top
J4  44,3.5 0 top
J6  12,49 0 top
J7  64.5,45.5 0 top
J8  64.5,12.5 0 top
J9  64.5,4 0 top
J10  64.5,33.5 0 top
J11  64.5,22 0 top
J12  44,46 0 top
J13  24.1,42.3 270 top
J14  3.5,46 0 top
J15  3.5,3.5 0 top
L1  18,25.8 0 top
R2  44.1,40.4 180 top
R3  23.96,47.64 90 top
R4  51,31.65 90 top
R5  51,22.5 90 top
R6  5.5,41 180 top
R7  2,33 180 top
R8  5.5,39 180 top
R9  2,35 180 top
R10  28.9,39.85 180 top
R11  28.9,41.6 180 top
R12  5.5,37 180 top
R13  55.25,18.75 0 top
R14  55.25,20.25 180 top
R18  35.1,21.8 90 top
R19  36.8,21.8 90 top
R20  38.5,21.8 90 top
R21  40.2,21.8 90 top
R24  49.02,40.55 0 top
R25  49.02,42.39 0 top
R26  31,21 0 top
R27  31,23 180 top
R28  48.25,30.15 90 top
R29  48.25,33.65 270 top
R31  31,17 0 top
R32  31,19 180 top
R33  48.25,20.5 90 top
R34  48.25,24.5 270 top
R36  31,13 0 top
R37  31,15 180 top
R38  31,9 0 top
R39  31,11 180 top
S1  11.9,2.8 180 top
S3  29.66,46.85 180 top
U1  13.9,34.1 180 top
U2  37.75,34.25 0 top
U$1  8,3.5 0 top
U$2  [CBA-SILK-LOGO]  17.1,2.8 0 top
U$3  48.5,3.5 0 top
U$4  2,41 0 top
U$5  2,39 0 top
U$8  2,37 0 top
U$9  57.25,41.75 180 top
U$10  57.25,33.25 180 top
U$11  57.25,25.25 180 top
U$14  27.3,7.3 90 bottom
Y1  14.8,27.1 0 top

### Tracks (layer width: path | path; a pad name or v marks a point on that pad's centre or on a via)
+3V3  (via drill 0.3, 0.35)
  Top 0.203: U2.P$24 32.36,29.5 v32.23,29.37 | R14.2 55,19.55 55,14.9 54.9,14.8 49.93,14.8 49.83,14.7 47.64,14.7 v47.43,14.9 | R10.2 26.53,41.27 26.53,41.63 24.56,43.6 22.2,43.6 22.1,43.6 | J3.2 23.06,30.6 v22,30.6
  Bottom 0.203: v32.23,29.37 30.76,27.9 25.76,27.9 J3.2 | v47.43,14.9 43.75,14.9 43.01,14.16 40.91,14.16 40.46,13.71 40.21,13.71 40.2,13.7 33.4,13.7 32.51,12.81 32.51,12.77 32.18,12.44 32.14,12.44 v31,11.3 | v22,30.6 22,28.8 v20.4,27.2
  pour Top: 22.5,50.5 22.5,24.5 33,24.5 33,-4.5 -2.5,-4.75 -3,50.5 arc-2
ATK0-CLKIN
  Top 0.152: U1.47 8.45,30.85 7.2,29.6 7.2,24.4 7.8,23.8 7.8,22.6 6.88,21.68 J1.P$1
ATK0-RX  (via drill 0.3)
  Top 0.152: U1.42 7.45,33.35 v7.4,33.3
  Bottom 0.152: J1.P$3 8,20.15 8,32.7 v7.4,33.3
ATK0-RXLED
  Top 0.152: R9.1 3.6,34.35 U1.40
ATK0-TX  (via drill 0.3)
  Top 0.152: U1.43 7.85,32.85 7.7,32.7 6.2,32.7 v5.7,33.2 | v4.9,21.7 4.9,21.6 3.5,20.2 3.5,17.52 J1.P$6
  Bottom 0.152: v5.7,33.2 4.9,32.4 4.9,31.6 6.3,30.2 6.3,25 4.6,23.3 4.6,22 v4.9,21.7
ATK0-TXLED
  Top 0.152: U1.41 3.8,33.85 R7.1
ATK-CLKOUT  (via drill 0.3)
  Top 0.152: U1.46 8.52,31.35 6.9,29.73 6.9,25.6 3.7,22.41 v3.7,21.7
  Bottom 0.152: v3.7,21.7 3.7,15.28 J1.P$8
CP1
  Top 0.203: U2.P$14 32.73,34.5 32.33,34.91 30.7,34.91 C19.1
CP2
  Top 0.203: U2.P$15 C19.2
DC-CAL  (via drill 0.3)
  Top 0.152: U2.P$12 32.77,35.5 32.63,35.64 32.6,35.64 v32.37,35.87 | v21,36.5 19.5,36.5 19.4,36.4 18.45,36.4 U1.13
  Bottom 0.152: v32.37,35.87 32.15,36.09 31.84,36.09 31.53,36.4 29.71,36.4 29.13,35.83 26.87,35.83 25.78,36.91 25.78,38.1 25.38,38.5 23,38.5 v21,36.5
DRV-HI-U  (via drill 0.35)
  Top 0.203: U2.P$47 44.3,36.5 44.77,36.97 44.77,38.03 44.94,38.2 45.31,38.2 v46.36,39.26
  Bottom 0.203: v46.36,39.26 46.68,39.26 47.1,39.67 47.19,39.67 R24.1
  other vias: 48.06,40.55
DRV-HI-V  (via drill 0.35)
  Top 0.203: U2.P$42 43.14,34 43.34,33.8 44.62,33.8 v44.75,33.67 | v46.9,32.3 46.9,30.55 R28.1
  Bottom 0.203: v44.75,33.67 46.12,32.3 v46.9,32.3
DRV-HI-W  (via drill 0.35)
  Top 0.203: U2.P$37 43.3,31.5 43.5,31.3 44.51,31.3 44.69,31.13 44.69,30.6 44.72,30.57 44.72,30.07 44.89,29.9 46.11,29.9 46.26,30.05 v46.51,30.05 | v46.12,28.78 46.3,28.6 46.62,28.6 47.8,27.42 47.8,26.3 47.61,26.1 47.52,26.1 47.34,25.93 47.34,20.45 R33.1
  Bottom 0.203: v46.51,30.05 46.51,29.17 v46.12,28.78
DRV-LO-U
  Top 0.203: U2.P$45 41.56,35.55 42.4,35.55 42.5,35.65 44.6,35.65 45.58,36.63 45.58,36.8 46.16,36.8 47.11,37.75 47.11,41.42 48.06,42.38 R25.1
DRV-LO-V
  Top 0.203: U2.P$40 42.99,33 43.01,32.98 43.97,32.98 44.32,32.63 45.18,32.63 47.15,34.6 R29.1
DRV-LO-W
  Top 0.203: U2.P$35 | U2.P$35 43.11,30.5 43.11,30.07 43.29,29.9 44.32,29.9 44.72,29.49 46.17,29.49 46.25,29.41 46.38,29.41 48.25,27.55 R34.1
DRV_EN  (via drill 0.3)  (1 unrouted)
  Top 0.152: U1.27 12.65,39.1 12.37,39.38 12.37,39.57 v12.14,39.8 | S3.P$4 S3.P$1
  Bottom 0.152: v12.14,39.8 12.35,39.8 12.68,40.13 13,40.13 14.47,41.6 21.17,41.6 23.47,43.91 24.51,43.91 26.05,45.45 31.95,45.45 v32,45.5
DRV_EN_DRV  (1 unrouted)
  Top 0.152: S3.P$2 S3.P$5 | U2.P$16 32.52,33.5 32.19,33.17 29.41,33.17 29.2,33.38 29.2,44.99
DRV_FAULT  (via drill 0.3)
  Top 0.152: U2.P$6 32.44,38.5 v32.36,38.58 | J13.1 23.2,42.3 22.2,41.3 21.17,41.3 20.68,40.81 16.52,40.81 15.69,39.98 15.62,39.98 14.65,39.01 U1.23
  Bottom 0.152: v32.36,38.58 32.24,38.7 30.36,38.7 29.26,37.6 29.26,37.24 28.76,36.74 27.24,36.74 26.7,37.29 26.7,41.07 25.48,42.28 24.12,42.28 J13.1
DRV_OCTW  (via drill 0.3)
  Top 0.152: U2.P$5 32.69,39 32.58,39.11 32.1,39.11 31.82,39.38 31.07,39.38 v30.84,39.61 | U1.26 13.15,39.35 v12.9,39.6
  Top 0.203: U2.P$5
  Bottom 0.152: v30.84,39.61 28.96,37.72 28.96,37.37 28.63,37.04 27.37,37.04 27,37.41 27,41.2 24.6,43.6 23.6,43.6 21.3,41.3 14.6,41.3 v12.9,39.6
ENC_CSN
  Top 0.152: U1.30 11.15,40.98 13.5,43.34 J6.5
ENC_MISO
  Top 0.152: U1.32 10.15,40.85 11.21,41.91 11.21,42.91 11.5,43.2 J6.3
ENC_MOSI  (via drill 0.3)
  Top 0.152: U1.33 9.5,37.95 v9.5,40.1
  Bottom 0.152: v9.5,40.1 13.62,44.23 J6.6
  other vias: 14.5,44.23
ENC_SCK
  Top 0.152: U1.31 10.65,40.92 12.5,42.77 J6.4
GND  (via drill 0.3, 0.35)  (6 unrouted)
  Top 0.152: U1.34 10.65,37.35 v11.5,36.5 | U1.24 14.15,37.35 15,36.5 v16,36.5 16.35,36.85 U1.14 | U1.60 15.65,31.65 v16,32 | U1.52 11.65,31.85 v11.5,32 11.15,32.35 U1.44 | R3.2 22.01,48.59 v22,48.6 | J6.1 9.5,43 C4.2
  Top 0.203: 39.15,35.08 v39.01,35.22 | U2.P$44 41.56,35.06 42.48,35.06 42.66,35.24 44.77,35.24 45.91,36.39 46.33,36.39 47.7,37.76 47.7,39.49 50.74,39.49 50.92,39.67 50.92,39.82 51.4,40.3 | 39.15,37.68 v39.01,37.82 | 39.15,28.98 v39.01,29.12 | C17.1 27.7,27.9 v27.7,28.85
  Bottom 0.203: 26,32.25 25.85,32.1 J3.1 22.4,32.1 22,32.5
  other vias: 36.47,37 37.74,37 39.01,37 36.47,36.11 36.47,35.22 36.47,34.33 36.47,32.56 36.47,33.45 36.47,31.67 37.74,36.11 37.74,35.22 39.01,36.11 39.01,34.33 37.75,34.25 37.74,33.45 37.74,32.56 37.74,31.67 39.01,33.45 39.01,32.56 39.01,31.67 28.4,38.4 28.4,37.6 28.5,29.65 55,44 54.3,44 50.3,17 48.7,28.2 45.05,40.4 44.9,39.1 48.9,36.2 48.9,37 49.1,46.9 49.1,46.1 43.2,26.5 43.2,25.7 43.2,24.8 28.3,19 31.95,19 31.95,23 28.3,23 28.3,15 28.3,11 31.95,11 31.95,15 27.95,41.6 36.47,39.6 37.74,39.6 39.01,39.6 36.47,38.71 36.47,37.82 37.74,38.71 37.74,37.82 39.01,38.71 36.47,30.9 37.74,30.9 39.01,30.9 36.47,30.01 36.47,29.12 37.74,30.01 37.74,29.12 39.01,30.01 36.07,42 36.07,42.8 36.07,43.8 36.07,44.6 39.77,46.1 40.27,48.1 37.97,48.1 37.57,46.2 35.67,48.1 35.07,46.2 33.87,48.1 33.87,46.2 33.87,43.6 30.77,43.1 28.37,46.8 35.97,26.62 35.97,25.82 37.77,26.62 34.37,25.82 55,43.2 54.3,43.2 55,42.4 54.3,42.4 55,41.6 54.3,41.6 55,40.8 54.3,40.8 53.2,44.7 51.1,44.7 48.5,44.7 49.7,43.9 52.2,43.1 51.1,41.7 53.2,41.7 52.2,40.7 51.1,29.1 51.9,29.1 52.7,29.1 50.3,29.1 49.5,29.1 49.5,28.3 50.3,28.3 51.1,28.3 51.9,28.3 52.7,28.3 49.9,27 52,27 53.7,28.7 51,27.4 49.6,20 50.4,20 51.2,20 52,20 52.8,20 52,19.2 52.8,19.2 51.2,19.2 50.4,19.2 49.6,19.2 48.1,18.4 48,15.9 49.7,15.9 49.6,18 52.8,18 52.8,15.9 54.2,15.9 54.2,18 52,17 27.7,29.65 28.5,28.85 27.6,37.6 27.6,38.4 6.45,41 7.75,38.3 8.9,42.4 13.5,34 5.6,31.9 15.2,40.7 18,43.5 18,45.2 18,47 20.1,35.7 18.7,27.3 14.8,27.1 9.85,2 14.96,17.15 10.2,27.4
  pour Top (no thermals): 40.5,25 34,25 34,41.25 33.5,41.5 26,41.5 26,50 43.5,50 43.5,45.5 38.5,45.5 38.55,41.5 41.75,41.5 41.5,41.25 41.5,35.5 40.25,35.5 40.25,34.5 40.5,34.5
  pour Bottom (rank 6): 33.5,-4 33.5,25 26,25 26,49.5 69,49.5 69.5,-4
  pour Bottom: 22.5,50 22.5,24.5 33,24.5 33,-4 -2,-4.25 -2,50
  pour Top (no thermals): 55.3,39.2 55.3,45.3 47.85,45.3 47.85,43.3 50.7,43.3 50.7,40 51.5,39.2
  pour Top (rank 2, no thermals): 49.4,29.8 52.6,29.8 52.8,30 53.3,30 54.4,28.9 54.4,28.2 54.2,28.2 54,28 52.5,26.5 50,26.5 49.9,26.5 47.8,28.6 47.8,29.5 48.1,29.8
  pour Top (no thermals): 48.4,20.7 52.7,20.7 53,20.8 55,20.8 55,14.9 47.6,14.9 47.6,19.9
  pour Bottom (rank 3, no thermals): 53.9,44.5 55.3,44.5 55.3,40 53.9,40
  pour Top (rank 3, no thermals): 42.8,26.8 42.8,24.9 42.6,24.7 42.6,24 43,24 43,21.4 42.9,21.3 41.3,21.3 41.3,19.9 43.7,19.9 43.9,20.1 43.9,26.8
I-V  (via drill 0.35)
  Top 0.152: U1.4 19.27,31.85 J3.3
  Top 0.203: U2.P$25 32.76,29 v32.23,28.47
  Bottom 0.203: v32.23,28.47 31.91,28.47 30.93,27.49 24.57,27.49 J3.3
I-W  (via drill 0.35)
  Top 0.152: U1.3 19.34,31.35 22.8,27.89 22.8,25.78 J3.4
  Top 0.203: U2.P$26 v35.17,28.5 | v35.17,28.5
  Bottom 0.203: v35.17,28.5 34.53,27.87 32.52,27.87 32.49,27.84 31.96,27.84 31.91,27.89 31.1,27.09 26.1,27.09 24.1,25.09 J3.4
M-GAIN  (via drill 0.3)
  Top 0.152: U2.P$10 32.18,36.5 v32.06,36.62 | v25.86,40.47 25.33,41 21.3,41 20.81,40.51 16.65,40.51 15.81,39.68 15.74,39.68 15.15,39.08 U1.22 15.2,38.65
  Bottom 0.152: v32.06,36.62 31.98,36.7 29.58,36.7 29.01,36.13 26.99,36.13 26.09,37.03 26.09,40.24 v25.86,40.47
M-PWM  (via drill 0.3)
  Top 0.152: U2.P$8 32.68,37.5 v32.36,37.82 | v20.95,35.74 20.73,35.52 20.73,35.12 20.59,34.99 19.6,34.99 19.47,35.12 19.47,35.63 19.25,35.85 U1.12
  Bottom 0.152: v32.36,37.82 31.78,38.4 30.49,38.4 29.57,37.47 29.57,37.12 28.88,36.43 27.12,36.43 26.39,37.16 26.39,40.69 26.08,41 23.5,41 22.4,39.9 22.4,38.4 21.03,37.03 20.78,37.03 20.47,36.72 20.47,36.28 20.73,36.02 20.73,35.97 v20.95,35.74
N$1  (via drill 0.3)
  Top 0.152: J1.YLWN 10.1,16.1 v8.6,14.6 | v2.7,29 1.05,30.65 R7.2
  Bottom 0.152: v8.6,14.6 8.6,11.1 7.5,10 5.3,10 2.4,12.9 2.4,22.2 4,23.8 4,27.7 v2.7,29
N$2  (via drill 0.35)
  Top 0.203: v51.8,39.68 52.33,39.45 52.58,39.45 52.78,39.25 U$9.GL
  Bottom 0.203: v51.8,39.68 51.78,39.7 50.92,39.7 50.77,39.85 50.77,40.81 49.97,41.61 R25.2
  other vias: 49.97,42.39
N$3  (via drill 0.35)
  Top 0.203: v50.13,40.55 R24.2 | U$9.GH 59.82,39.18 59.88,39.18 60.06,39 60.06,38.4 59.88,38.22 59.12,38.22 58.74,38.6 55.76,38.6 55.38,38.22 54.62,38.22 54,38.84 50.92,38.84 v50.9,38.86
  Bottom 0.203: v50.13,40.55 50.13,39.91 50.61,39.43 50.61,39.15 v50.9,38.86
N$4
  Top 0.203: U$10.GH 59.82,30.68 59.88,30.68 60.06,30.5 60.06,29.9 59.88,29.72 59.12,29.72 58.64,30.2 55.86,30.2 55.38,29.72 54.48,29.72 53.53,30.67 51.6,30.67 51.05,30.68 50.82,30.91 49.45,30.91 49.2,30.67 48.68,30.67 R28.2
N$5
  Top 0.203: U$11.GH 59.82,22.68 59.88,22.68 60.06,22.5 60.06,21.9 59.88,21.72 59.12,21.72 58.74,22.1 55.7,22.1 55.56,21.95 55.56,21.9 55.38,21.72 50.86,21.72 50.82,21.76 50.3,21.76 50.25,21.72 49.92,21.72 | 49.92,21.72 | R33.2 49.13,21.45 49.4,21.72 49.92,21.72
N$6
  Top 0.203: U$11.GL 54.68,22.68 54.62,22.68 54.07,22.13 51.03,22.13 50.99,22.17 50.13,22.17 50.08,22.13 49.67,22.13 R34.2
N$7
  Top 0.203: U2.P$38 43.38,32 43.66,31.71 44.67,31.71 45.09,31.3 45.09,31.01 C33.1
N$8
  Top 0.203: U2.P$43 C32.1 | C32.1
N$9
  Top 0.203: U2.P$48 43.45,37 C31.1
N$10
  Top 0.203: U2.P$55 | U2.P$55 42.6,40.5 42.7,40.4 R2.2
N$11
  Top 0.203: U2.P$27 | U2.P$27 33,28 32.85,27.85 C20.2
N$12
  Top 0.152: Y1.1 14.37,27.62 14.37,27.95 14.65,28.22 U1.58
N$13
  Top 0.203: U2.P$33 41.45,29.45 40.32,29.45 39.2,28.33 39.2,26.73 39.28,26.65 39.28,26.16 38.51,25.39 38.42,25.31 37.61,25.31 37.29,24.99 36.05,24.99 C28.1 35.1,23.95 R18.2
N$14
  Top 0.203: U2.P$32 41.44,28.95 40.39,28.95 39.61,28.16 39.61,26.9 39.69,26.82 39.69,25.91 38.58,24.91 37.77,24.91 36.97,24.1 C28.2 36.95,22.9 R19.2
N$15
  Top 0.203: U2.P$31 41.44,28.45 40.47,28.45 40.01,27.99 40.01,27.07 40.09,26.99 40.09,25.74 C29.1 38.35,22.9 R20.2
N$16
  Top 0.203: U2.P$30 40.6,28 40.42,27.82 40.42,27.23 40.5,27.16 40.5,24.35 C29.2 40.25,22.8 R21.2
N$17
  Top 0.152: U1.59 15.15,28.02 15.23,27.95 15.23,27.62 Y1.3
N$18  (1 unrouted)
  Top 0.203: U2.P$13 32.81,35 32.5,35.31 31.79,35.31 C13.2
N$19
  Top 0.203: U2.P$49 42.5,37.5 43.2,38.2 43.2,39 C8.1
N$20
  Top 0.203: U2.P$11 34.84,36 35.08,35.77 35.08,30.23 34.84,30 U2.P$23 31.9,30 30.9,29 | C17.2 30.9,29 | 30.9,29 C14.2
N$21
  Top 0.203: U2.P$7 | R11.1 30.11,41.44 34.9,41.44 35.08,41.27 35.08,38.23 35,38.16 35,38 U2.P$7
N$22
  Top 0.152: J1.GRNN 8.49,10.49 8,10 5.3,10 2.4,12.9 2.4,22.2 4,23.8 4,28.7 1.8,30.9 1.8,34.25 R9.2
N$23
  Top 0.152: R12.2 U$8.2
N$24
  Top 0.203: U$10.GL 54.03,30.75 53.69,31.08 51.22,31.08 50.99,31.32 49.63,31.32 R29.2
N$25
  Top 0.152: R10.1 30.62,39.08 31.7,39.08 31.83,38.95 31.83,37.6 32.43,37 U2.P$9
  Top 0.203: 29.85,39.55 R10.1
N$26
  Top 0.152: R3.1 25.6,46.69 27.06,48.14 | 27.06,48.14 S3.P$6 | S3.P$3 27.16,48.04 27.06,48.14
N$27  (via drill 0.3)
  Top 0.152: U1.56 13.65,28.7 13.02,28.07 13.02,24.36 13.99,23.38 v13.99,22.8
  Bottom 0.152: v13.99,22.8 19.99,22.8 J2.1
  other vias: 20.04,22.85
N$28  (via drill 0.3)
  Top 0.152: U1.57 14.15,28.77 13.32,27.95 13.32,24.49 J2.5 14.96,18.93 13.99,17.97 v13.99,17.5 | S1.P$4 v14.22,7.97
  Bottom 0.152: v13.99,17.5 14.22,17.27 v14.22,7.97
N$34
  Top 0.152: U1.62 16.65,29.05 17.1,28.6 C12.1 17.05,27.25 L1.1
N$35
  Top 0.152: R6.2 U$4.2
N$36
  Top 0.152: R8.2 U$5.2
PHASE-U  (via drill 0.3, 0.35)  (1 unrouted)
  Top 0.203: U2.P$46 41.56,36.05 44.43,36.05 45.17,36.8 45.17,37.12 C31.2 45.55,37.55 v46.4,38.4 | U$9.SH 59.82,39.68 60.38,39.68 60.56,39.5 60.56,38.32 60.05,37.81 58.95,37.81 58.58,38.19 55.92,38.19 55.55,37.81 54.45,37.81 53.83,38.44 51.37,38.44 51.16,38.23 50.64,38.23 50.03,38.83 48.36,38.83 v48.33,38.86 48.33,38.43 48.11,38.21 48.11,37.6 46.56,36.05 v46.56,34.91
  Bottom 0.152: 35.59,17.01 31.95,20.64 R26.2
  Bottom 0.203: v48.33,38.86 46.86,38.86 v46.4,38.4 | v46.56,34.91 46.04,34.91 45.81,35.13 45.29,35.13 44.12,33.96 44.12,33.41 45,32.53 45,31.5 44.73,31.23 43.64,31.23 43.27,30.86 43.27,30.34 43.48,30.12 43.48,29.34 43.26,29.12 43.26,28.59 43.91,27.95 43.91,19.08 41.83,17.01 35.59,17.01
  other vias: 59.6,44 60.3,44 59.6,43.2 60.3,43.2 59.6,42.4 60.3,42.4 59.6,41.6 60.3,41.6 59.6,40.8 60.3,40.8 61.4,44 62.1,42.7 63.7,42 65.9,41.9 67.5,42.6 61.3,46.4 61.4,41.6 61.7,39.9 63.8,40.2 66,40.3 31.95,21
  pour Top (rank 3, no thermals): 59.3,40.2 59.3,45.2 62.7,48.7 62.7,49.5 68.5,49.5 68.5,39.1 61,39.1 61,39.8 60.5,40.2
  pour Bottom (rank 3, no thermals): 59.3,39.1 59.3,45.2 62.7,48.7 62.7,49.5 68.5,49.5 68.5,39.1
PHASE-V  (via drill 0.3, 0.35)  (1 unrouted)
  Top 0.203: U2.P$41 43.06,33.5 43.17,33.39 44.14,33.39 44.49,33.04 45.01,33.04 45.38,33.41 45.38,34.33 C32.2 | U$10.SH 59.82,31.18 60.38,31.18 60.56,31 60.56,29.82 60.05,29.31 58.95,29.31 58.48,29.79 56.02,29.79 55.55,29.31 54.31,29.31 53.36,30.26 51.34,30.26 v50.56,30.28
  Bottom 0.152: 34.84,15.97 32.98,15.97 R31.2 | 48.5,29.83 49.32,29.83 49.47,29.68 49.96,29.68 v50.56,30.28
  Bottom 0.203: v50.56,30.28 50.56,33.07 49.96,33.67 49.44,33.67 49.21,33.44 46.61,33.44 C32.2 | 48.5,29.83 47.16,28.48 47.16,28.35 45.13,26.32 45.13,18.58 42.34,15.79 37.5,15.79 37.43,15.72 37.43,15.71 37.06,15.34 36.46,15.34 35.83,15.97 34.84,15.97
  other vias: 45.55,34.5 59.5,35.5 60.2,35.5 59.5,34.7 60.2,34.7 59.5,33.9 60.2,33.9 59.5,33.1 60.2,33.1 59.5,32.3 60.2,32.3 61.3,35.5 61.2,32.3 61.2,33.9 63,36.9 63.5,29.9 61.8,31.1 64.5,37.4 65.6,29.6 66.5,37.3 67,30 62.8,37.9 62.9,28.8 31.95,17
  pour Bottom (rank 3): 68.5,38.6 62.2,38.6 62.2,36.1 59.3,36.1 59.2,36 59.2,30.5 62.2,30.5 62.2,28.3 68.5,28.3
  pour Top (rank 3, no thermals): 68.5,38.6 59.2,38.6 59.2,31.7 60.5,31.7 61,31.2 61,29.6 60.3,28.9 59.2,28.9 59.2,28.4 59.3,28.3 68.5,28.3
PHASE-W  (via drill 0.3, 0.35)  (1 unrouted)
  Top 0.203: U2.P$36 | C33.2 43.6,30.9 43.33,30.9 43.22,31 U2.P$36 | U$11.SH 59.82,23.18 60.38,23.18 60.56,23 60.56,21.82 60.05,21.31 58.95,21.31 58.58,21.69 55.92,21.69 55.55,21.31 50.74,21.31 v50.56,21.13 | v46.2,26.1 46.2,27 45.46,27.74 45.32,27.74 44.21,28.86 v43.89,28.86
  Bottom 0.152: 34.67,15.56 32.11,13 R36.2
  Bottom 0.203: v43.89,28.86 43.89,30.59 C33.2 | v50.56,21.13 49.8,21.89 49.8,23.09 50.33,23.62 50.33,24.15 49.96,24.52 47.78,24.52 v46.2,26.1 45.8,26.1 45.53,25.83 45.53,18.41 42.5,15.38 37.68,15.38 37.23,14.93 36.3,14.93 35.66,15.56 34.67,15.56
  other vias: 43.9,30.6 59.6,27.4 60.3,27.4 59.6,26.6 60.3,26.6 59.6,25.8 60.3,25.8 59.6,25 60.3,25 59.6,24.2 60.3,24.2 61.5,27.4 61.6,25.5 61.6,23.5 63,27.4 63,25.8 63.1,24.6 64.5,27.4 64.5,25.8 66,25.8 66,27.4 66.5,24.6 67.6,18.3 31.95,13
  pour Top (rank 3, no thermals): 59.3,27.8 68.5,27.8 68.5,17.8 63.5,17.8 61,20.3 61,23.3 60.6,23.7 59.3,23.7
  pour Bottom (rank 3, no thermals): 68.5,27.8 59.3,27.8 59.3,22 63.5,17.8 68.5,17.8
PWMHIU  (1 unrouted)
  Top 0.152: 15.67,38.62 15.7,38.65 15.7,39.2 15.87,39.37 15.94,39.37 16.77,40.2 21.23,40.2 21.67,39.76 J13.2 25.54,39.76 26.9,38.4 26.9,35.25 29.28,32.87 32.32,32.87 32.45,33 U2.P$17
PWMHIV  (2 unrouted)
  Top 0.152: 23.35,37.22 22.13,38.43 20.97,39.59 17.03,39.59 16.65,39.22 U1.19 | U2.P$19 32.47,32 32.21,32.26 29.03,32.26 26.29,34.99 26.29,36.61 25.7,37.2 24.12,37.2
PWMHIW
  Top 0.152: U1.17 18.04,38.99 20.71,38.99 22.4,37.3 22.4,36.67 24.1,34.97 J13.4 24.12,34.66 25.76,34.66 | U2.P$21 32.6,31 31.95,31.65 28.77,31.65 25.76,34.66 | 25.76,34.66 25.74,34.68
PWMLOU
  Top 0.152: U1.20 16.15,39.15 16.9,39.9 21.1,39.9 22.5,38.5 25.9,38.5 26.59,37.8 26.59,35.12 29.15,32.56 32.34,32.56 32.4,32.5 U2.P$18
PWMLOV  (1 unrouted)
  Top 0.152: U2.P$20 32.54,31.5 32.09,31.95 28.9,31.95 25.99,34.87 25.99,35.41 25.4,36 23.5,36 22.7,36.8 22.7,37.44 20.85,39.29 17.39,39.29 17.15,39.05
PWMLOW
  Top 0.152: U2.P$22 32.67,30.5 31.83,31.34 28.65,31.34 26.59,33.4 23.7,33.4 22.8,34.3 22.8,35.84 22.09,36.55 22.09,37.18 20.59,38.68 19.23,38.68 U1.16
SHNT-V-HI  (via drill 0.35)
  Top 0.203: v35.1,16.6 R18.1
  Bottom 0.203: R4.SB 48.34,33.04 47.53,32.23 47.53,32.04 44.52,29.03 44.52,28.59 44.31,28.39 44.31,18.91 42,16.6 v35.1,16.6
  other vias: 49.7,33.04
SHNT-V-LO  (via drill 0.35)
  Top 0.203: v36.8,15.97 R19.1
  Bottom 0.203: R4.SA 48.34,30.24 46.75,28.65 46.75,28.52 44.72,26.49 44.72,18.75 42.17,16.19 37.03,16.19 v36.8,15.97
  other vias: 49.7,30.24
SHNT-W-HI  (via drill 0.35)
  Top 0.203: v38.5,14.75 R20.1
  Bottom 0.203: v38.5,14.75 38.73,14.97 42.67,14.97 45.94,18.24 45.94,22.74 47.09,23.89 R5.SB
  other vias: 49.7,23.89
SHNT-W-LO  (via drill 0.35)
  Top 0.203: v40.2,14.34 R21.1
  Bottom 0.203: R5.SA 49.7,21.41 49.39,21.72 49.39,22.19 48.1,23.48 47.25,23.48 46.34,22.57 46.34,18.07 42.84,14.57 40.4,14.57 40.2,14.37 v40.2,14.34
  other vias: 49.7,21.09
SL-V  (via drill 0.35)
  Top 0.203: U2.P$39 42.6,32.5 42.69,32.59 42.8,32.59 42.82,32.58 43.8,32.58 44.15,32.23 45.35,32.23 47.07,33.95 48.98,33.95 49.48,34.45 R4.B
  other vias: 54.3,35.5 55,35.5 54.3,34.7 55,34.7 54.3,33.9 55,33.9 54.3,33.1 55,33.1 54.3,32.3 55,32.3
  pour Top (no thermals): 49.4,35.4 52.6,35.4 53.8,36.6 53.9,36.6 55.3,36.6 55.4,36.5 55.4,31.3 55.4,31.2 55.3,31.1 49.4,31.1
  pour Bottom (rank 3, no thermals): 55.3,36 55.3,31.5 53.9,31.5 53.9,36
SL-W  (via drill 0.35)
  Top 0.203: U2.P$34 41.56,29.95 42.67,29.95 43.12,29.49 44.15,29.49 45.49,28.15 46.18,28.15 v47.17,27.16 | 50.26,25.73 50.67,25.73 | 51,25.73 50.67,25.73 | 50.67,25.73 50.45,25.95 | 50.45,25.95 50.3,26.1 | v48.88,26.8 48.88,26.42 49.35,25.95 50.45,25.95
  Bottom 0.203: v48.88,26.8 47.53,26.8 v47.17,27.16
  other vias: 55,27.5 54.3,27.5 55,26.7 54.3,26.7 55,25.9 54.3,25.9 55,25.1 54.3,25.1 55,24.3 54.3,24.3
  pour Top (no thermals): 55.3,28 54.2,28 52.4,26.2 47.5,26.2 47.5,22.8 49,21.3 54.4,21.3 55.3,22.2
  pour Bottom (rank 3, no thermals): 55.3,28 53.9,28 53.9,23.5 55.3,23.5
STLCLK
  Top 0.152: U1.37 8.53,35.85 8.37,35.69 6.49,35.69 5.87,36.3 5.87,37.7 6.45,38.27 R8.1
STLERR
  Top 0.152: U1.36 8.6,36.35 8.24,35.99 7.26,35.99 7.12,36.12 7.12,36.33 R12.1
THERMISTOR
  Top 0.203: R14.1 R13.2
V-U
  Top 0.152: R27.2 R26.1 D7.1 26.7,22.65 C39.1 | U1.2 19.41,30.85 22.49,27.76 22.49,25.65 22.8,25.35 22.8,23.24 J3.5
  Top 0.203: 26.55,22.85 C39.1 25.64,21.94 J3.5
  Bottom 0.203: 24.1,22 J3.5
V-V
  Top 0.152: R32.2 R31.1 D2.1 26.7,18.65 C41.1 | U1.1 19.48,30.35 22.19,27.64 22.19,25.51 22.49,25.2 22.49,23.11 22.8,22.81 22.8,20.7 J3.6
  Top 0.203: C41.1 24.5,19 J3.6
V-VCC
  Top 0.152: R39.2 R38.1 D5.1 26.7,10.65 C45.1 | U1.63 17.15,29.05 17.3,28.9 20.06,28.9 21.58,27.38 21.58,25.26 21.89,24.95 21.89,22.86 22.19,22.56 22.19,20.45 22.49,20.14 22.49,18.03 22.8,17.73 22.8,15.62 J3.8
  Top 0.203: C45.1 24.1,13.6 J3.8
V-W
  Top 0.152: R37.2 R36.1 D3.1 26.7,14.65 C43.1 | U1.64 19.8,29.6 21.89,27.51 21.89,25.38 22.19,25.08 22.19,22.99 22.49,22.68 22.49,20.57 22.8,20.27 22.8,18.16 J3.7
  Top 0.203: C43.1 25.96,15 J3.7
VCC  (via drill 0.35)
  Top 0.152: R38.2 33.9,9
  other vias: 56.9,35.5 57.2,20.9 56.2,35.5 57.6,35.5 58.3,35.5 56.9,27.5 56.2,27.5 57.6,27.5 58.3,27.5 56.9,44 56.2,44 57.6,44 58.3,44 56.9,34.7 56.2,34.7 57.6,34.7 58.3,34.7 56.9,26.7 56.2,26.7 57.6,26.7 58.3,26.7 56.9,43.2 56.2,43.2 57.6,43.2 58.3,43.2 56.9,33.9 56.2,33.9 57.6,33.9 58.3,33.9 56.9,25.9 56.2,25.9 57.6,25.9 58.3,25.9 56.9,42.4 56.2,42.4 57.6,42.4 58.3,42.4 56.9,33.1 56.2,33.1 57.6,33.1 58.3,33.1 56.9,25.1 56.2,25.1 57.6,25.1 58.3,25.1 56.9,41.6 56.2,41.6 57.6,41.6 58.3,41.6 56.9,32.3 56.2,32.3 57.6,32.3 58.3,32.3 56.9,24.3 56.2,24.3 57.6,24.3 58.3,24.3 56.9,40.8 56.2,40.8 57.6,40.8 58.3,40.8 58.2,20.9 57.2,20 58.2,20 59.2,20.4 60,19.6 57.2,19 58.2,19 57.2,18 58.2,18 59.2,18.5 60.9,18.5 56.4,15.3 58.5,16 60.4,16.6 62.2,17.3 56.5,45.7 58,45.7 59.2,46.9 55,46.9 57.2,46.9 53.8,48.4 56.2,48.4 58.3,48.4 60.7,48.4 63.4,16.6 61.3,15.8 59.4,15 57.6,14.9 56.5,28.4 57.9,28.4 57.2,29 56.5,23.5 57.9,23.5 57.2,22.9 56.5,36.3 57.9,36.3 57.2,37.2 56.5,31.5 57.9,31.5 57.2,31 56.5,40 57.9,40 57.2,39.4 52.7,46.6 51.4,48.4
  pour Top (rank 5, no thermals): 26,50.5 26,25 33.5,25 33.5,-4.5 70,-4.5 69.5,50.5
  pour Bottom (rank 4): 55.4,45.3 55.3,15.8 55.3,9.7 60.1,9.7 63.2,8.5 68.5,8.6 68.5,17.6 63.4,17.6 59.2,21.8 59.1,28.1 59.3,28.3 61.9,28.3 61.9,30.1 61.8,30.2 59.3,30.2 59.1,30.4 59.1,36.2 59.3,36.4 61.9,36.4 61.9,38.6 59.3,38.6 59.1,38.8 59.1,45.4 62.5,48.8 62.5,49.5 49.7,49.5 49.8,45.3

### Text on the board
tPlace: < no - go > | SPI | FAULT | U | HI1 | HI2 | HI3 | GND | V | 3V3 | I-V | W | I-W | V-U | V-V | V-W | VCC | UP0 | V-VCC | ATKP0 | atkbldcdriver v0.5 | GND
bPlace: since systems tend to leave unstable equilibria / they cannot often be in them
